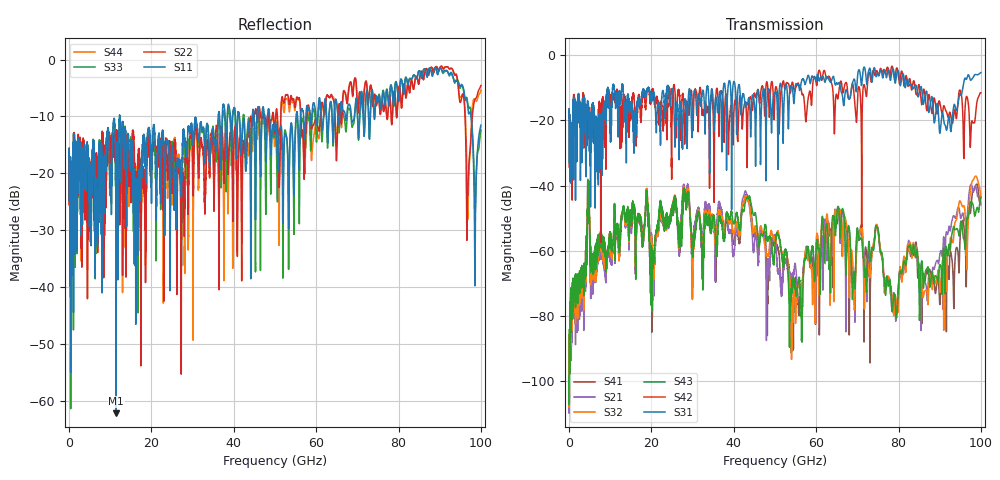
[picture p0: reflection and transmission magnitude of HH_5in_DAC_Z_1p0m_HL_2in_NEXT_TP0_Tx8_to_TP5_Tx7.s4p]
# GHz S RI R 45
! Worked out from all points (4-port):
!   4000 points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, 25 MHz to 100 GHz, reference 45 ohm
!   strongest paths, dB at 25 MHz, 25.02 GHz, 50.02 GHz, 75.03 GHz, 100 GHz:
!     S31: -18.8, -10.2, -11.4, -5.7, -5.3
!     S42: -18.8, -19.7, -11.3, -5.7, -11.5
!     S43: -98.4, -48.1, -57.9, -53.3, -43.7
!     S32: -99.9, -47.2, -58.4, -53.8, -43.6
!     S21: -101.4, -47.4, -55.8, -53.3, -45.9
!     S41: -99.9, -48.2, -58.7, -53.9, -43.4
!   lowest |S11| = -62.1 dB at 11.43 GHz (marker M1), VSWR 1.00, Z = 45 - j0.0645 ohm
!   |S11| at or under -10 dB: start of sweep to 12.26 GHz; 12.4 GHz to 36.22 GHz (23.82 GHz wide, 98 % of centre); 48.71 GHz to 55.13 GHz (6.426 GHz wide, 12.4 % of centre)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
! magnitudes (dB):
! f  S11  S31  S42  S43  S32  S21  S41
! 25 MHz  -17.1  -18.8  -18.8  -98.4  -99.9  -101.4  -99.9
! 11.43 GHz  -62.1  -16.0  -13.6  -54.3  -54.7  -55.7  -55.3
! 43.2 GHz  -15.2  -14.8  -29.8  -43.9  -43.9  -43.1  -43.0
! 54.23 GHz  -13.0  -10.1  -8.3  -70.4  -88.3  -69.4  -80.6
! 65.58 GHz  -11.2  -8.4  -10.5  -48.0  -47.7  -49.7  -47.1
! 79.1 GHz  -5.1  -7.9  -7.5  -73.9  -75.2  -76.0  -73.4
! 100 GHz  -11.5  -5.3  -11.5  -43.7  -43.6  -45.9  -43.4
